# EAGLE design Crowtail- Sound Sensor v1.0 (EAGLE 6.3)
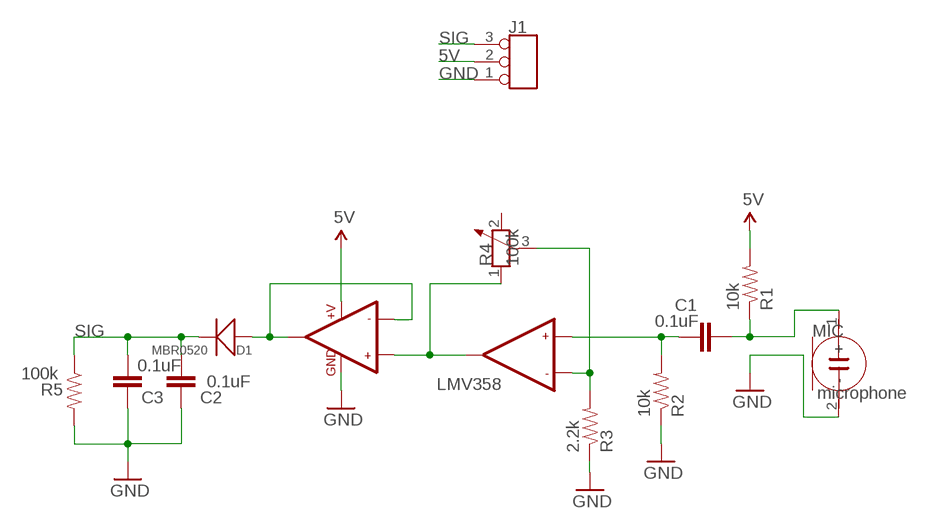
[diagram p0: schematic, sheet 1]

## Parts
C1  0.1uF  CAP0603-CAP  [0603-CAP]
C2  0.1uF  CAP0603-CAP  [0603-CAP]
C3  0.1uF  CAP0603-CAP  [0603-CAP]
D1  MBR0520  D'MBR0520LT1'  [SOD123-2.7X1.6]
J1  TINKER_3P_DIP  [3P_2.0_DIP]
MIC  microphone  MICROPHONE  [2P-D8.9MM]
R1  10k  RESISTOR0603-RES  [0603-RES]
R2  10k  RESISTOR0603-RES  [0603-RES]
R3  2.2k  RESISTOR0603-RES  [0603-RES]
R4  100k  R-POTENTIOMETER'3362'  [3P-SQUA-7X6.8]
R5  100k  RESISTOR0603-RES  [0603-RES]
U1  LMV358  [SO08]

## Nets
5V: J1.2 R1.2 U1.8(+V)
GND: C2.1 C3.1 J1.1 MIC.2(-) R2.1 R3.1 R5.2 U1.4(GND)
N$6: C1.1 MIC.1(+) R1.1
N$8: R3.2 R4.3 U1.6(-IN2)
N$11: C1.2 R2.2 U1.5(+IN2)
N$13: D1.2(+) U1.1(OUT1) U1.2(-IN1)
N$16: R4.1 U1.3(+IN1) U1.7(OUT2)
SIG: C2.2 C3.2 D1.1(-) J1.3 R5.1
Unconnected: R4.2

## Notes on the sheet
- LMV358

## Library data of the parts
C1-C3 = SparkFun:CAP: Capacitor
D1 = Discrete:D*
J1 = Connector:TINKER_3P_DIP
MIC = template:MICROPHONE
R1-R3 R5 = SparkFun:RESISTOR: Resistor
R4 = Discrete:R-POTENTIOMETER*: Potentiometer
U1 = SparkFun:LMV358

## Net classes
0 default: width 0.203 mm
1 power: width 0.254 mm

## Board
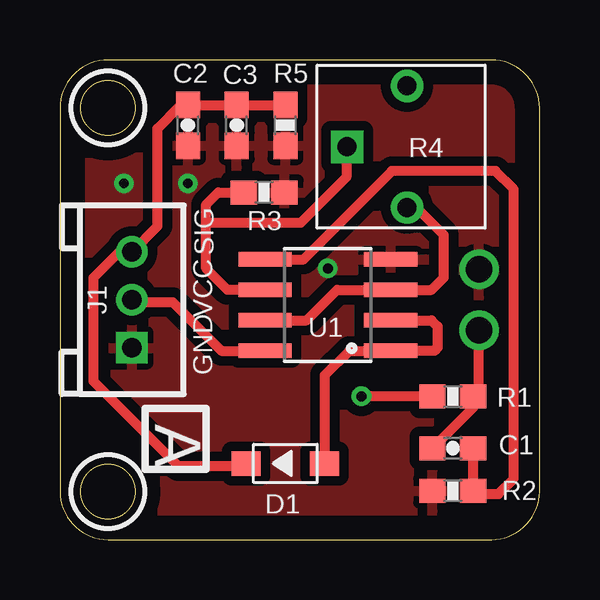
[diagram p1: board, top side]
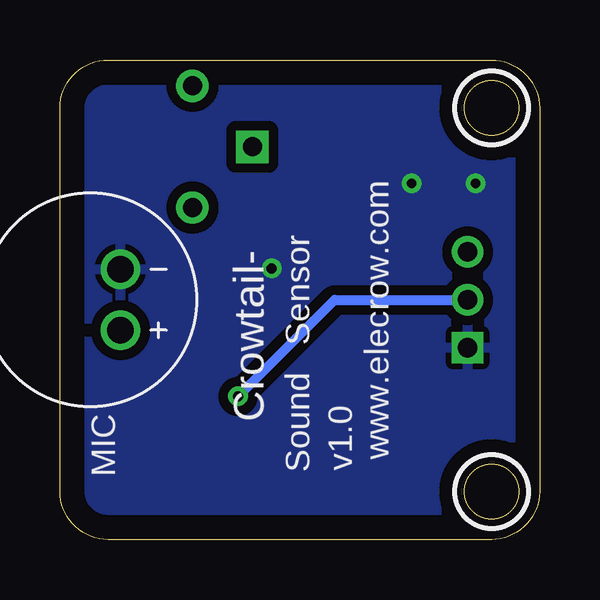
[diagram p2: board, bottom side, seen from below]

Size 20 x 20 mm. Coordinates in mm from the lower left corner, seen from the top.
Outline: 20,2 20,18 arc90 18,20 2,20 arc90 0,18 0,2 arc90 2,0 18,0 arc90 20,2
Outline: circle at 2,18 radius 1.14
Outline: circle at 2,2 radius 1.14
Copper layers (1*16): Top 0.035mm / dielectric 1.5mm / Bottom 0.035mm
Design rules "default *": minimum track width 10mil, minimum drill 24mil, track to track 8mil, track to pad 8mil, pad to pad 8mil, via to via 8mil, smd to smd 8mil, copper to edge 40mil, drill to drill 8mil, minimum pad ring 10mil, minimum via ring 8mil, stop-mask expansion 2mil, vias tented up to drill 100mil, thermal gap 10mil
tRestrict: area 0.5,16.5 to 3.5,19.5; area 0.5,0.5 to 3.5,3.5
bRestrict: area 0.5,16.5 to 3.5,19.5; area 0.5,0.5 to 3.5,3.5

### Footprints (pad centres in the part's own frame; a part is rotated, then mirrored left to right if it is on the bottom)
0603-CAP = smd 1.1 x 1: 1 -0.85,0; 2 0.85,0
SOD123-2.7X1.6 = smd 1.2 x 1.02: 1 1.635,0; 2 -1.635,0
3P_2.0_DIP = drill 0.8 pad 1.27 square: 1 -2,0 | drill 0.8 pad 1.27: 2 0,0; 3 2,0
2P-D8.9MM = drill 1.1: 1 -1.27,1.27; 2 -1.27,-1.27
0603-RES = smd 1.1 x 1: 1 -0.85,0; 2 0.85,0
3P-SQUA-7X6.8 = drill 0.8 pad 1.35: 1 -2.54,-0.25; 2 2.54,-0.25 | drill 0.8 pad 1.35 square: 3 0,2.25
SO08 = smd 0.61 x 2.21: 1 -1.905,-2.616; 2 -0.635,-2.616; 3 0.635,-2.616; 4 1.905,-2.616; 5 1.905,2.616; 6 0.635,2.616; 7 -0.635,2.616; 8 -1.905,2.616

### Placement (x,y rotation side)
C1  16.38,3.81 0 top
C2  5.33,17.27 90 top
C3  7.37,17.27 90 top
D1  9.4,3.17 180 top
J1  3,10 90 top
MIC  18.75,10 180 bottom
R1  16.38,5.97 180 top
R2  16.38,2.03 0 top
R3  8.51,14.48 180 top
R4  14.22,16.38 90 top
R5  9.4,17.27 270 top
U1  11.18,9.78 90 top

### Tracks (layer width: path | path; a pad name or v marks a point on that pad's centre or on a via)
5V  (via drill 0.41)
  Top 0.406: J1.2 3.09,9.91 4.7,9.91 6.73,7.87 U1.8 | R1.2 v12.57,5.97
  Bottom 0.406: J1.2 8.54,10 v12.57,5.97
GND  (via drill 0.41 pad 0.51)
  other vias: 5.33,14.86 2.67,14.86 11.18,11.3
  pour Top (isolate 0.406): -1.27,20.32 20.32,20.32 20.32,0 -1.27,0
  pour Bottom (isolate 0.406): -1.27,20.32 20.32,20.32 20.32,0 -1.27,0
N$6
  Top 0.406: MIC.1 17.48,6.21 R1.1 17.23,5.51 C1.1
N$8
  Top 0.406: U1.6 6.99,10.41 6.1,11.3 6.1,13.21 | 6.1,13.21 6.1,13.97 6.6,14.48 R3.2 | R4.3 11.94,16.35 11.94,15.11 10.03,13.21 6.1,13.21
N$11
  Top 0.406: U1.5 10.16,11.68 13.84,15.37 18.16,15.37 18.92,14.61 18.92,2.54 18.29,1.91 17.36,1.91 R2.2 C1.2
N$13
  Top 0.406: U1.2 15.49,9.14 15.75,8.89 15.75,8 15.62,7.87 U1.1 12.06,7.87 11.05,6.86 11.05,3.19 D1.2
N$16
  Top 0.406: R4.1 14.86,13.84 16,12.7 16,10.92 15.49,10.41 U1.3 11.56,10.41 10.29,9.14 U1.7
SIG
  Top 0.406: R5.1 C3.2 C2.2 5.04,18.12 4.06,17.14 4.06,13.06 J1.3 2.48,12 1.4,10.92 1.4,6.6 4.95,3.05 7.64,3.05 D1.1

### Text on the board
tPlace: SIG | VCC | GND | A
bPlace: www.elecrow.com | Sensor | Crowtail- | Sound | v1.0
